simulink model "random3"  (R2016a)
settings: Solver=VariableStepDiscrete  StartTime=0.0  StopTime=1e4  RelTol=1e-3
StopFcn:
  | plot_random3(random3out)
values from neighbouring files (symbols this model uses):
  high = str2double(get_param('random3/Bereichszaehler', 'high'))    [plot_random3.m]
  low = str2double(get_param('random3/Bereichszaehler', 'low'))    [plot_random3.m]
libraries: simulink x1

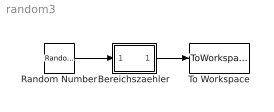
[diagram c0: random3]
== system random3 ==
  Bereichszaehler : Subsystem
  Random Number : RandomNumber  Mean=100  Variance=10  SampleTime=1  VectorParams1D=off
  To Workspace : ToWorkspace  VariableName=random3out  SaveFormat=Structure With Time  SampleTime=-1
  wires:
  Random Number/1 -> Bereichszaehler/1(In)
  Bereichszaehler/1(Anteil) -> To Workspace/1

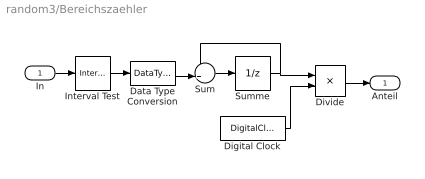
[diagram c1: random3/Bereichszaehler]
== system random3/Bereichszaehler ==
  In : Inport
  Data Type Conversion : DataTypeConversion  OutDataTypeStr=double
  Digital Clock : DigitalClock
  Divide : Product  Inputs=*/
  Interval Test : simulink/Logic and Bit Operations/Interval Test  IntervalClosedRight=on  uplimit=(low+step):step:high  IntervalClosedLeft=off  lowlimit=low:step:(high-step)  OutDataTypeStr=uint8
  Sum : Sum  Inputs=++|
  Summe : UnitDelay  SampleTime=-1
  Anteil : Outport
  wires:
  Data Type Conversion/1 -> Sum/2
  Interval Test/1 -> Data Type Conversion/1
  Digital Clock/1 -> Divide/2
  Divide/1 -> Anteil/1
  In/1 -> Interval Test/1
  Summe/1 -> Divide/1, Sum/1
  Sum/1 -> Summe/1
